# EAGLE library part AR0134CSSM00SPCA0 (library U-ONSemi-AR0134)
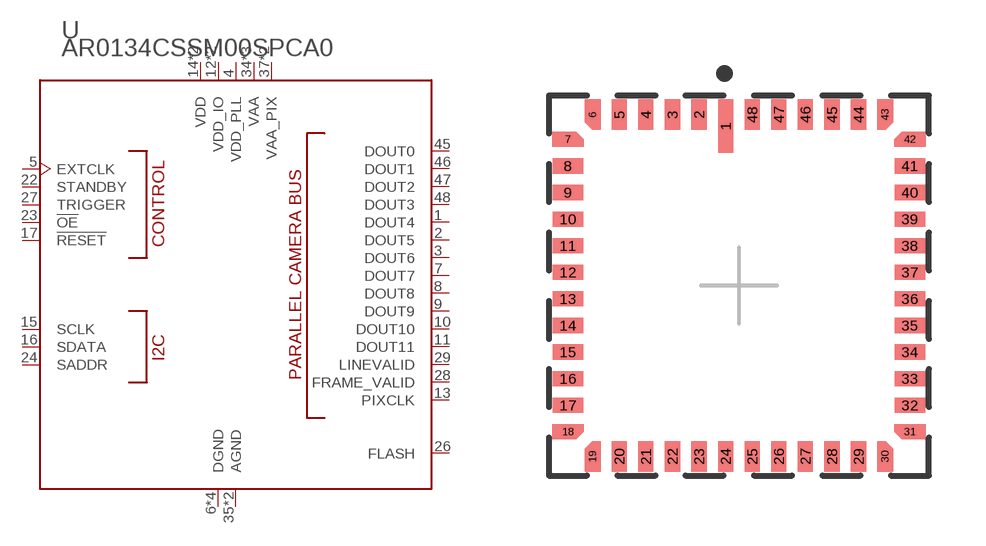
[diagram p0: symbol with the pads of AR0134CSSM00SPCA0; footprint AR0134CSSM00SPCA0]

Designator prefix U

## AR0134CSSM00SPCA0  [AR0134CSSM00SPCA0]
1  DOUT4
2  DOUT5
3  DOUT6
4  VDD_PLL  pwr
5  EXTCLK
6  DGND  pwr
7  DOUT7
8  DOUT8
9  DOUT9
10  DOUT10
11  DOUT11
12  VDD_IO  pwr
13  PIXCLK
14  VDD  pwr
15  SCLK
16  SDATA
17  !RESET
18  VDD_IO  pwr
19  VDD  pwr
22  STANDBY
23  !OE
24  SADDR
25  DGND  pwr
26  FLASH
27  TRIGGER
28  FRAME_VALID
29  LINEVALID
30  DGND  pwr
34  VAA  pwr
35  AGND  pwr
36  VAA  pwr
37  VAA_PIX  pwr
38  VAA_PIX  pwr
39  AGND  pwr
40  VAA  pwr
44  DGND  pwr
45  DOUT0
46  DOUT1
47  DOUT2
48  DOUT3

## Footprint AR0134CSSM00SPCA0 (pad centres in mm)
smd 0.4 x 1.4: 1 -0.35,4.2
smd 0.4 x 0.8: 2 -1.05,4.5; 3 -1.75,4.5; 4 -2.45,4.5; 5 -3.15,4.5; 20 -3.15,-4.5; 21 -2.45,-4.5; 22 -1.75,-4.5; 23 -1.05,-4.5; 24 -0.35,-4.5; 25 0.35,-4.5; 26 1.05,-4.5; 27 1.75,-4.5; 28 2.45,-4.5; 29 3.15,-4.5; 44 3.15,4.5; 45 2.45,4.5; 46 1.75,4.5; 47 1.05,4.5; 48 0.35,4.5
smd 0.3 x 0.5: 6 -3.85,4.5; 19 -3.85,-4.5; 30 3.85,-4.5; 43 3.85,4.5
smd 0.5 x 0.3: 7 -4.5,3.85; 18 -4.5,-3.85; 31 4.5,-3.85; 42 4.5,3.85
smd 0.8 x 0.4: 8 -4.5,3.15; 9 -4.5,2.45; 10 -4.5,1.75; 11 -4.5,1.05; 12 -4.5,0.35; 13 -4.5,-0.35; 14 -4.5,-1.05; 15 -4.5,-1.75; 16 -4.5,-2.45; 17 -4.5,-3.15; 32 4.5,-3.15; 33 4.5,-2.45; 34 4.5,-1.75; 35 4.5,-1.05; 36 4.5,-0.35; 37 4.5,0.35; 38 4.5,1.05; 39 4.5,1.75; 40 4.5,2.45; 41 4.5,3.15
